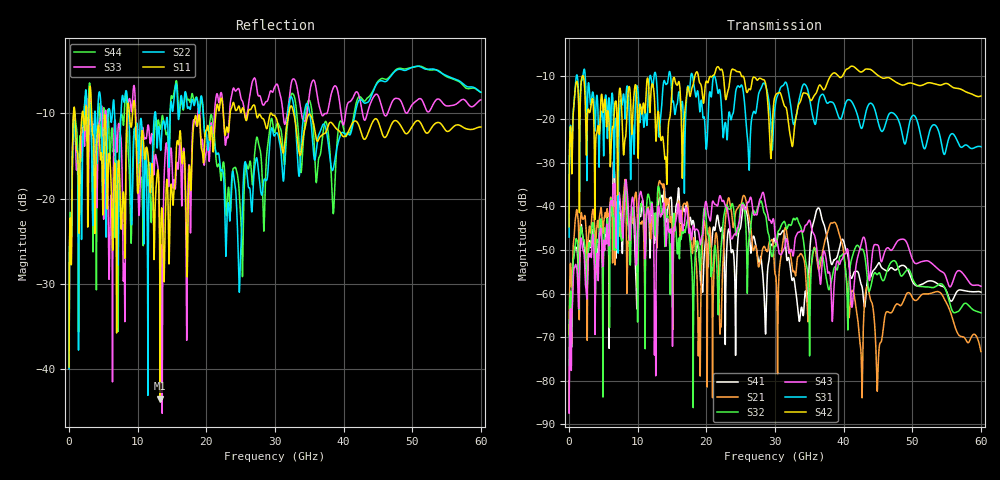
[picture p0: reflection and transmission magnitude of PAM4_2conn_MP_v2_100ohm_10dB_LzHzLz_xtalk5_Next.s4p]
! Info: Touchstone file created by Circ.  Input file=FAB50GbE_2conn_Midplane_Examax_Topo2_v2_100ohm_10dB_LzHzLz.circ
# Hz S RI R 50
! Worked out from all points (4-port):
!   6000 points, 10 MHz to 60 GHz, reference 50 ohm
!   strongest paths, dB at 10 MHz, 15.01 GHz, 30.01 GHz, 45.01 GHz, 60 GHz:
!     S42: -44.7, -13.0, -14.7, -9.9, -14.7
!     S31: -47.0, -15.4, -17.2, -20.6, -26.3
!     S43: -87.5, -51.5, -46.4, -48.9, -58.3
!     S32: -69.8, -52.5, -49.1, -55.5, -64.4
!     S21: -69.3, -45.1, -55.4, -77.7, -73.3
!     S41: -87.2, -41.6, -48.0, -53.2, -59.7
!   lowest |S11| = -43.5 dB at 13.27 GHz (marker M1), VSWR 1.01, Z = 49.4 + j0.126 ohm
!   |S11| at or under -10 dB: 3.275 GHz to 8.452 GHz (5.177 GHz wide, 88.3 % of centre); 9.649 GHz to 21.39 GHz (11.74 GHz wide, 75.6 % of centre); 32.74 GHz to end of sweep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
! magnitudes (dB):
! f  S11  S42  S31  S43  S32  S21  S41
! 10 MHz  -39.8  -44.7  -47.0  -87.5  -69.8  -69.3  -87.2
! 2.07 GHz  -10.1  -10.1  -9.5  -50.3  -47.6  -42.8  -47.4
! 13.27 GHz  -43.5  -23.3  -20.9  -42.1  -37.7  -34.3  -37.9
! 18.95 GHz  -10.2  -11.2  -16.8  -46.7  -51.4  -65.7  -51.0
! 25.49 GHz  -9.7  -10.5  -15.0  -40.2  -39.9  -37.5  -39.7
! 28.56 GHz  -11.2  -11.4  -12.0  -38.8  -41.8  -49.5  -66.4
! 60 GHz  -11.6  -14.7  -26.3  -58.3  -64.4  -73.3  -59.7
